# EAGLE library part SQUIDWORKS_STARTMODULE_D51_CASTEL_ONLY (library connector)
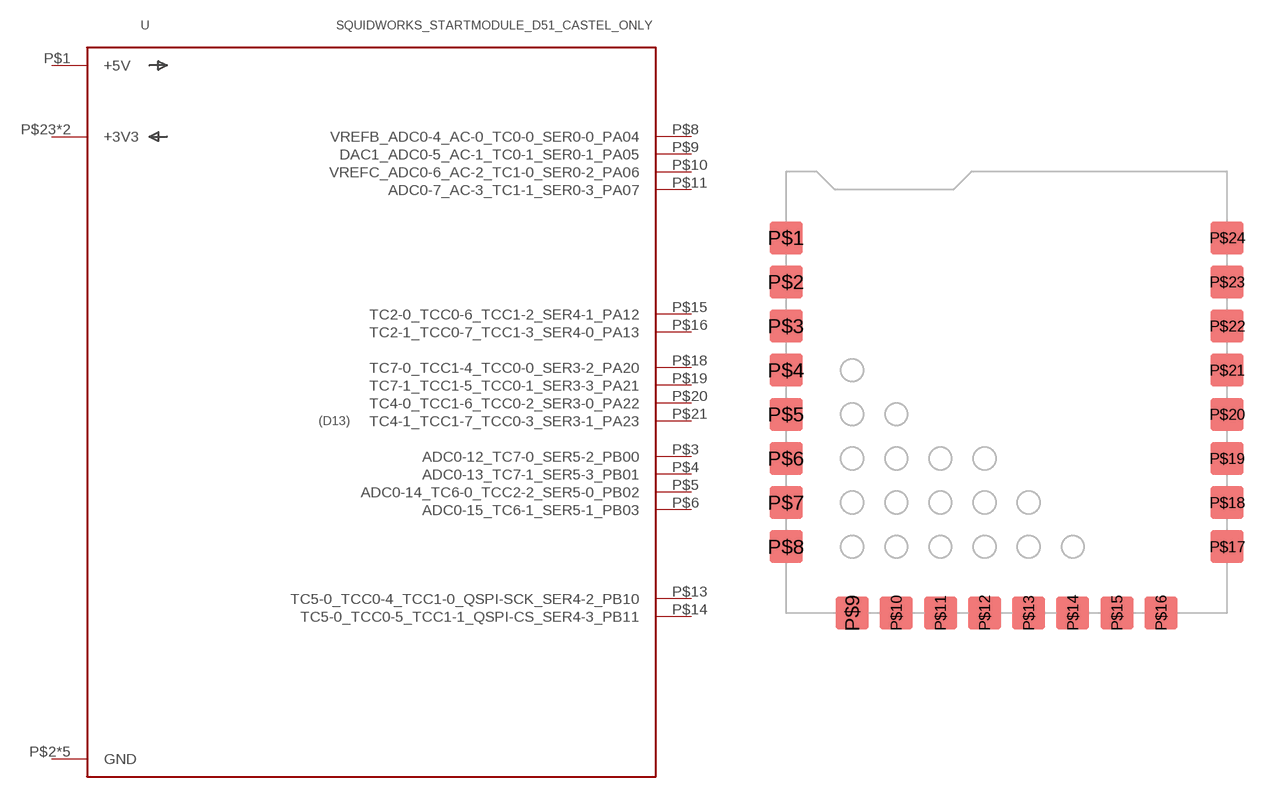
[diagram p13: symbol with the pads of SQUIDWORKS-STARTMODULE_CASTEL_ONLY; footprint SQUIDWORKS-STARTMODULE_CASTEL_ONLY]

Designator prefix U

## SQUIDWORKS_STARTMODULE_D51_CASTEL_ONLYCO  [SQUIDWORKS-STARTMODULE_CASTEL_ONLY]
P$1  +5V
P$2  GND
P$3  ADC0-12_TC7-0_SER5-2_PB00
P$4  ADC0-13_TC7-1_SER5-3_PB01
P$5  ADC0-14_TC6-0_TCC2-2_SER5-0_PB02
P$6  ADC0-15_TC6-1_SER5-1_PB03
P$7  GND
P$8  VREFB_ADC0-4_AC-0_TC0-0_SER0-0_PA04
P$9  DAC1_ADC0-5_AC-1_TC0-1_SER0-1_PA05
P$10  VREFC_ADC0-6_AC-2_TC1-0_SER0-2_PA06
P$11  ADC0-7_AC-3_TC1-1_SER0-3_PA07
P$12  GND
P$13  TC5-0_TCC0-4_TCC1-0_QSPI-SCK_SER4-2_PB10
P$14  TC5-0_TCC0-5_TCC1-1_QSPI-CS_SER4-3_PB11
P$15  TC2-0_TCC0-6_TCC1-2_SER4-1_PA12
P$16  TC2-1_TCC0-7_TCC1-3_SER4-0_PA13
P$17  GND
P$18  TC7-0_TCC1-4_TCC0-0_SER3-2_PA20
P$19  TC7-1_TCC1-5_TCC0-1_SER3-3_PA21
P$20  TC4-0_TCC1-6_TCC0-2_SER3-0_PA22
P$21  TC4-1_TCC1-7_TCC0-3_SER3-1_PA23
P$22  GND
P$23  +3V3
P$24  +3V3

## Footprint SQUIDWORKS-STARTMODULE_CASTEL_ONLY (pad centres in mm)
smd 1.905 x 1.905: P$1 -12.7,8.89; P$2 -12.7,6.35; P$3 -12.7,3.81; P$4 -12.7,1.27; P$5 -12.7,-1.27; P$6 -12.7,-3.81; P$7 -12.7,-6.35; P$8 -12.7,-8.89; P$9 -8.89,-12.7; P$10 -6.35,-12.7; P$11 -3.81,-12.7; P$12 -1.27,-12.7; P$13 1.27,-12.7; P$14 3.81,-12.7; P$15 6.35,-12.7; P$16 8.89,-12.7; P$17 12.7,-8.89; P$18 12.7,-6.35; P$19 12.7,-3.81; P$20 12.7,-1.27; P$21 12.7,1.27; P$22 12.7,3.81; P$23 12.7,6.35; P$24 12.7,8.89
